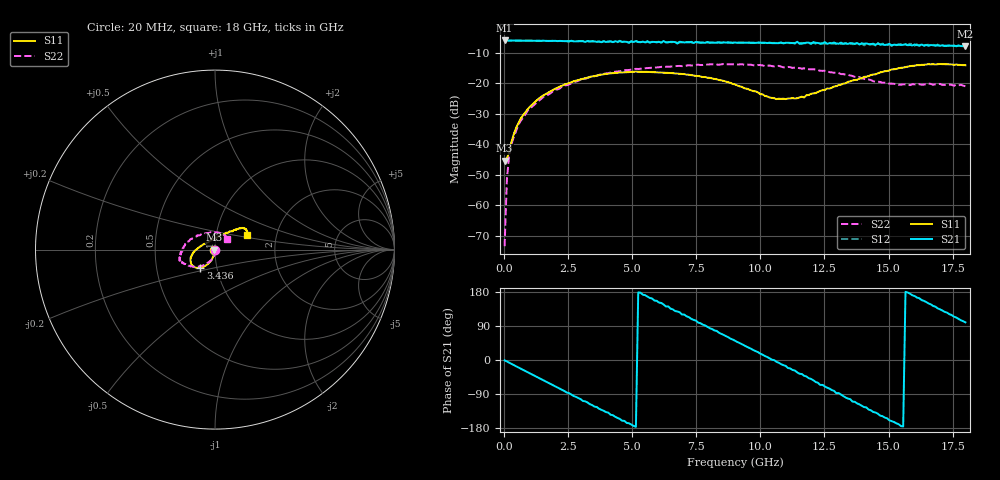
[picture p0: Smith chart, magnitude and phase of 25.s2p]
!Agilent Technologies,N5230A,US43500223,A.07.50.48
!Agilent N5230A: A.07.50.48
!Date: Monday, February 01, 2016 11:57:18
!Correction: S11(Full 2 Port(1,2))
!S21(Full 2 Port(1,2))
!S12(Full 2 Port(1,2))
!S22(Full 2 Port(1,2))
!S2P File: Measurements: S11, S21, S12, S22:
# Hz S  RI  R 50
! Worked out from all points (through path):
!   201 points, 20 MHz to 18 GHz, reference 50 ohm
!   highest |S21| = -5.93 dB at 20 MHz (marker M1); lowest = -7.8 dB at 18 GHz (marker M2)
!   group delay of S21, straight-line fit = 95.5 ps
!   lowest |S11| = -45.4 dB at 20 MHz (marker M3), VSWR 1.01, Z = 49.5 - j0.0661 ohm
!   |S11| at or under -10 dB: start of sweep to end of sweep
!   |S22| runs from -73.4 to -13.7 dB; largest |S21 - S12| = 0.032
!   S11 on the Smith chart (normalised r, x): 20 MHz: 0.99, -0.00; 3.436 GHz: 0.83, -0.17; 18 GHz: 1.41, +0.25
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2e7  -0.00534 -0.000668  0.5049 -0.00661  0.5047 -0.00712  7.02e-05 -0.000202
1.099e8  -0.00533 -0.00271  0.5027 -0.035  0.5026 -0.0352  0.00108 -0.00247
1.998e8  -0.00413 -0.00612  0.4999 -0.0635  0.4995 -0.0629  0.00111 -0.00668
3.796e8  -0.00457 -0.014  0.4886 -0.1173  0.4885 -0.1178  0.00135 -0.0131
5.594e8  -0.00527 -0.0217  0.4726 -0.1697  0.472 -0.1706  0.000218 -0.0208
9.19e8  -0.00889 -0.0367  0.4237 -0.2672  0.4229 -0.2682  -0.00487 -0.0353
1.4584e9  -0.0191 -0.0576  0.3149 -0.3852  0.3133 -0.3866  -0.0176 -0.0534
2.1776e9  -0.0387 -0.0795  0.1226 -0.4817  0.1195 -0.4804  -0.0398 -0.0726
3.0766e9  -0.069 -0.097  -0.1534 -0.4671  -0.1487 -0.4691  -0.0735 -0.0908
3.4362e9  -0.0823 -0.1007  -0.2389 -0.4306  -0.2416 -0.4215  -0.0891 -0.0959
4.9645e9  -0.1256 -0.089  -0.4836 -0.0826  -0.4847 -0.0629  -0.1416 -0.0904
6.0433e9  -0.1357 -0.0663  -0.4218 0.2283  -0.4157 0.2386  -0.1654 -0.0798
7.4817e9  -0.128 -0.0318  -0.1164 0.4631  -0.0971 0.4602  -0.187 -0.0715
9.01e9  -0.0958 0.00745  0.2955 0.3623  0.2988 0.3557  -0.197 -0.0553
1.05383e10  -0.0391 0.0415  0.457 -0.00265  0.4607 -0.019  -0.1884 -0.0189
1.14373e10  -0.0107 0.0559  0.4045 -0.2592  0.3817 -0.253  -0.18 0.00771
1.20666e10  0.0113 0.0673  0.2824 -0.3816  0.2582 -0.3816  -0.1674 0.0302
1.3505e10  0.0599 0.0898  -0.1055 -0.4457  -0.1213 -0.4316  -0.1156 0.0696
1.50333e10  0.1172 0.1131  -0.4154 -0.1586  -0.4077 -0.1445  -0.0325 0.0935
1.64717e10  0.1661 0.1175  -0.3784 0.1932  -0.3846 0.1888  0.0385 0.089
1.73707e10  0.1797 0.0988  -0.2131 0.354  -0.2031 0.3705  0.0614 0.0733
1.8e10  0.1793 0.0841  -0.0661 0.3998  -0.0451 0.4066  0.0685 0.0573
